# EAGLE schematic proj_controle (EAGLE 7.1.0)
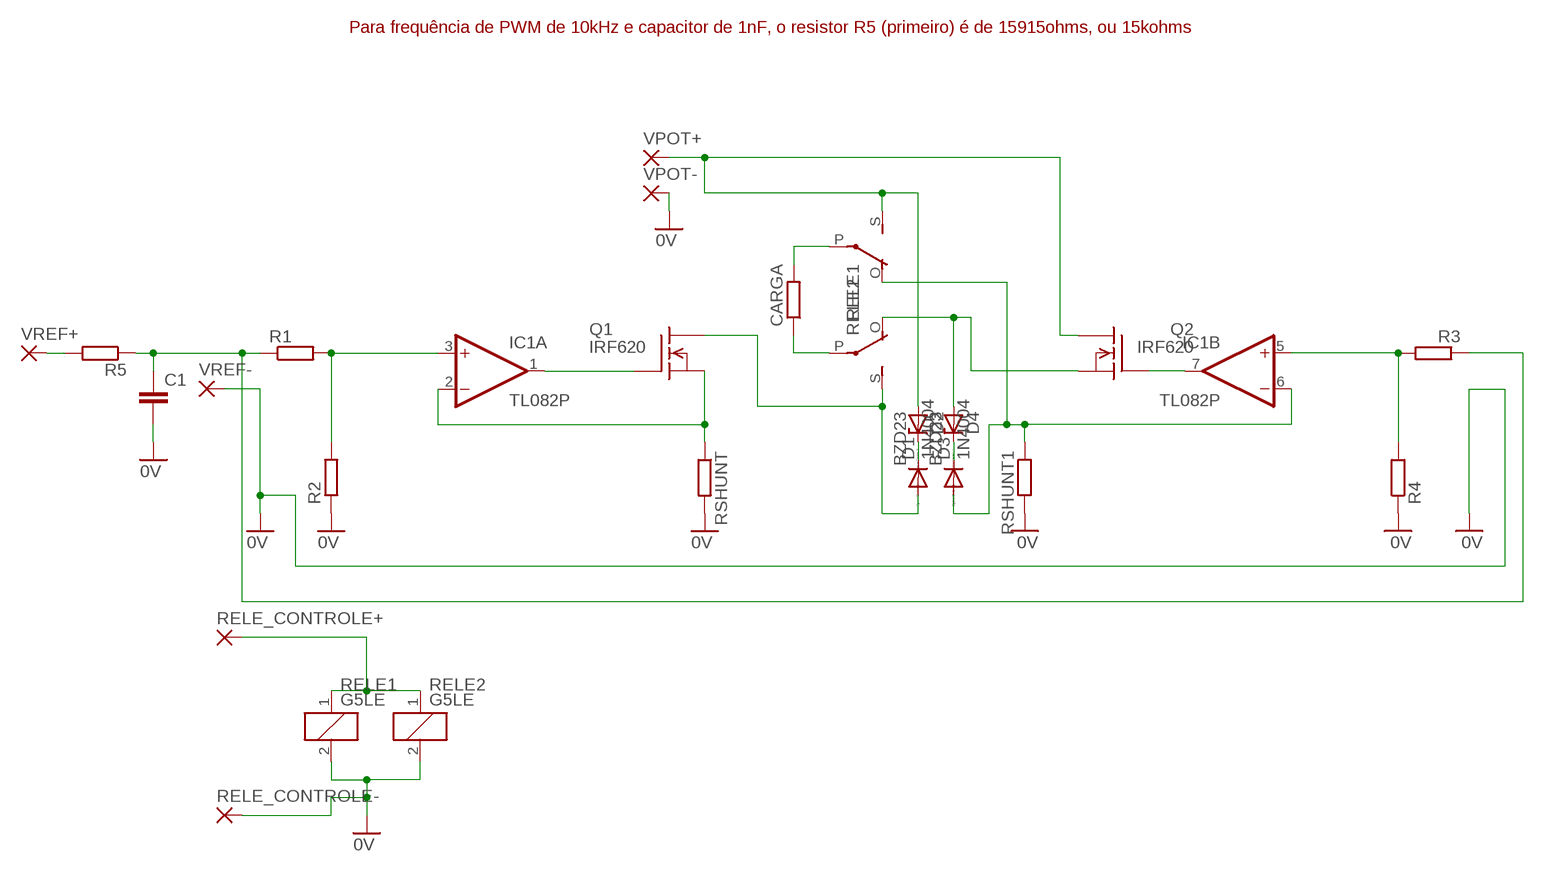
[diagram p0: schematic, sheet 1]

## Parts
C1  C-EU050-025X075  [C050-025X075]
CARGA  R-EU_0207/10  [0207/10]
D1  1N4004  [DO41-10]
D2  BZD23  [SOD81]
D3  1N4004  [DO41-10]
D4  BZD23  [SOD81]
IC1  TL082P  [DIL08]
Q1  IRF620  [TO220]
Q2  IRF620  [TO220]
R1  R-EU_0207/10  [0207/10]
R2  R-EU_0207/10  [0207/10]
R3  R-EU_0207/10  [0207/10]
R4  R-EU_0207/10  [0207/10]
R5  R-EU_0207/10  [0207/10]
RELE1  G5LE  [G5LE]
RELE2  G5LE  [G5LE]
RELE_CONTROLE+  3,17/1,1  [3,17/1,1]
RELE_CONTROLE-  3,17/1,1  [3,17/1,1]
RSHUNT  R-EU_0617/22  [0617/22]
RSHUNT1  R-EU_0617/22  [0617/22]
VPOT+  3,17/1,1  [3,17/1,1]
VPOT-  3,17/1,1  [3,17/1,1]
VREF+  3,17/1,1  [3,17/1,1]
VREF-  3,17/1,1  [3,17/1,1]

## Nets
0V: C1.2 R2.1 R4.1 RELE1.2 RELE2.2 RELE_CONTROLE-.1(P) RSHUNT1.2 RSHUNT.2 VPOT-.1(P) VREF-.1(P)
N$1: CARGA.1 RELE2.P(2:P)
N$2: IC1.3(A:+IN) R1.2 R2.2
N$3: IC1.1(A:OUT) Q1.1(G)
N$4: IC1.2(A:-IN) Q1.3(S) RSHUNT.1
N$5: C1.1 R1.1 R3.1 R5.1
N$6: R5.2 VREF+.1(P)
N$7: CARGA.2 RELE1.P(2:P)
N$8: D1.A Q1.2(D) RELE2.S(2:S)
N$9: IC1.5(B:+IN) R3.2 R4.2
N$10: IC1.7(B:OUT) Q2.1(G)
N$11: D3.A IC1.6(B:-IN) RELE1.O(2:O) RSHUNT1.1
N$12: D1.C D2.C
N$13: D2.A Q2.2(D) RELE1.S(2:S) VPOT+.1(P)
N$14: D4.A Q2.3(S) RELE2.O(2:O)
N$15: RELE1.1 RELE2.1 RELE_CONTROLE+.1(P)
N$16: D3.C D4.C

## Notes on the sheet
- Para frequência de PWM de 10kHz e capacitor de 1nF, o resistor R5 (primeiro) é de 15915ohms, ou 15kohms

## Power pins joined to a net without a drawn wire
V+: IC1.8(P:V+)
V-: IC1.4(P:V-)

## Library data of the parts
C1 = rcl:C-EU: CAPACITOR, European symbol
CARGA R1-R5 = rcl:R-EU_: RESISTOR, European symbol
D1 D3 = diode:1N4004: DIODE
D2 D4 = diode:BZD23: Z DIODE
IC1 = linear:TL082: OP AMP Data sheet; DATA_SHEET: <a href="http://www.ti.com/lit/ds/symlink/tl084a.pdf"> Data sheet </a>
Q1 Q2 = transistor-fet:IRF620: N-Channel Enhancement MOSFET (HEXFET); 200V; 5,2A; 0,8Ohm
RELE1 RELE2 = relay:G5LE: RELAY 1 x switch, 10 A/120 V AC, 8 A/30 V DC, Omron; OC_FARNELL: unknown; OC_NEWARK: unknown
RELE_CONTROLE+ RELE_CONTROLE- VPOT+ VPOT- VREF+ VREF- = wirepad:3,17/1,1: THROUGH-HOLE PAD
RSHUNT RSHUNT1 = resistor:R-EU_: RESISTOR, European symbol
